(* Logix 5000 AddOnInstructionDefinition export DCO_ReadDriveParameter; software revision 20.01 *)

ADD_ON_INSTRUCTION DCO_ReadDriveParameter   (* revision 1.0 *)
VAR_INPUT
   Parameter_Value : INT; {visible}
   Instance_Number_Read : INT; {visible}
   Attribute_Number_Read : INT; {visible}
END_VAR
VAR_IN_OUT
   MSG_IN : MESSAGE; {required}
END_VAR
VAR_INPUT
   Value_Out_Read : INT; {access None}
END_VAR

ROUTINE Logic   (* ladder *)
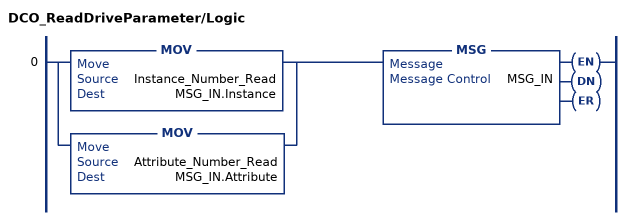
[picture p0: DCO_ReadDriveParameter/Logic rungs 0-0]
   0: [MOV(Instance_Number_Read,MSG_IN.Instance) ,MOV(Attribute_Number_Read,MSG_IN.Attribute) ]MSG(MSG_IN);
END_ROUTINE
END_ADD_ON_INSTRUCTION
